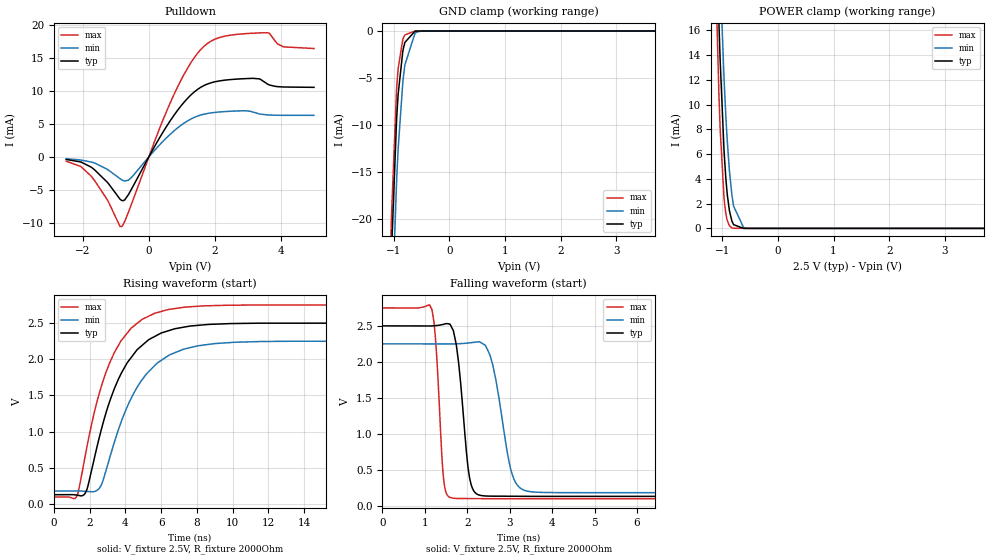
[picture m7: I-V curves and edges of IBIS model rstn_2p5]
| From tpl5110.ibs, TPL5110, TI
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|   Model
[Model]   rstn_2p5
Model_type   I/O_open_drain
Polarity   Non-Inverting
Enable   Active-Low
Vinl = 0.75
Vinh = 1.75
Vmeas = 1.25
Vref = 2.5
Cref = 1pF
Rref = 2000
|   typ   min   max
C_comp   0.474pF   0.343pF   0.582pF
[Voltage Range]   2.5   2.25   2.75
[Temperature Range]   25   105   -40
[Pullup Reference]   2.5   2.25   2.75
[Pulldown Reference]   0   0   0
[Power Clamp Reference]   2.5   2.25   2.75
[GND Clamp Reference]   0   0   0
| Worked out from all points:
|   slope of the pulldown table from 0 to 0.375 V, typ, clamps not added: 113 ohm
|   GND clamp passes 1 mA (typ) near -0.77 V on its own axis
|   POWER clamp passes 1 mA (typ) near -0.85 V on its own axis
|   falling waveform, V_fixture 2.5V, R_fixture 2000Ohm: 20-80 % time 217ps typ, 346ps min, 145ps max; typ from 2.5 V to 0.13 V
|   rising waveform, V_fixture 2.5V, R_fixture 2000Ohm: 20-80 % time 2.09ns typ, 2.26ns min, 1.95ns max; typ from 0.13 V to 2.5 V
[Pulldown]
|   Voltage   I(typ)   I(min)   I(max)
-2.5V     -377.8uA   -275.3uA   -643.7uA
-1.75V    -1.525mA   -756.3uA   -2.874mA
-827.5mV  -6.561mA   -3.438mA   -10.54mA
-512.5mV  -4.763mA   -3.037mA   -6.974mA
747.5mV   6.204mA    3.877mA    9.293mA
1.235V    9.192mA    5.639mA    13.95mA
1.67V     10.81mA    6.471mA    16.74mA
2.217V    11.57mA    6.84mA     18.18mA
3.147V    11.9mA     6.802mA    18.73mA
3.605V    10.99mA    6.358mA    18.79mA
4.077V    10.59mA    6.301mA    16.66mA
5V        10.54mA    6.298mA    16.41mA
[GND Clamp]
|   Voltage   I(typ)   I(min)   I(max)
-2.5V     -532.7mA   -498.3mA   -571.1mA
-1.045V   -24.97mA   -32.7mA    -21.13mA
-1.038V   -23.46mA   -31.2mA    -19.56mA
-947.5mV  -9.534mA   -16.15mA   -6.257mA
-940mV    -8.737mA   -15.16mA   -5.592mA
-917.5mV  -6.657mA   -12.44mA   -3.935mA
-835mV    -2.176mA   -5.473mA   -895.3uA
-820mV    -1.735mA   -4.645mA   -662.1uA
-797.5mV  -1.211mA   -3.602mA   -417uA
-617.5mV  -27.18uA   -264uA     -5.53uA
-512.5mV  -1.678uA   -25.84uA   -162.4nA
5V        0A         0A         0A
[POWER Clamp]
|   Voltage   I(typ)   I(min)   I(max)
-2.5V     351.8mA    332.8mA    370.5mA
-1.15V    31.09mA    37.5mA     25.49mA
-1.06V    16.49mA    23.38mA    10.69mA
-1.038V   13.47mA    20.27mA    7.946mA
-962.5mV  5.816mA    11.51mA    2.17mA
-910mV    2.716mA    7.028mA    631.3uA
-872.5mV  1.433mA    4.681mA    212.1uA
-827.5mV  591.6uA    2.703mA    43.28uA
-797.5mV  301.6uA    1.804mA    12.76uA
-617.5mV  1.108uA    70.67uA    0A
-565mV    156.4nA    19.84uA    0A
5V        0A         0A         0A
[Ramp]
R_load = 2000
|   typ   min   max
dV/dt_r   1.42208/2.09402e-09   1.24152/2.26178e-09   1.59152/1.95148e-09
dV/dt_f   1.42208/2.17249e-10   1.24152/3.46422e-10   1.59152/1.454e-10
[Falling Waveform]
V_fixture = 2.5V
V_fixture_min = 2.25V
V_fixture_max = 2.75V
R_fixture = 2000Ohm
C_fixture = 0F
|   Time   V(typ)   V(min)   V(max)
0s        2.5V       2.25V      2.75V
1.167ns   2.499V     2.249V     2.723V
1.281ns   2.505V     2.249V     2.05V
1.446ns   2.522V     2.249V     346.2mV
1.694ns   2.368V     2.249V     102.3mV
2.064ns   357mV      2.265V     99.11mV
2.428ns   135.2mV    2.228V     97.83mV
3.075ns   131.4mV    406mV      97.51mV
3.575ns   130mV      189.6mV    97.51mV
50ns      129.9mV    180.8mV    97.47mV
[Rising Waveform]
V_fixture = 2.5V
V_fixture_min = 2.25V
V_fixture_max = 2.75V
R_fixture = 2000Ohm
C_fixture = 0F
|   Time   V(typ)   V(min)   V(max)
0s        129.9mV    180.8mV    97.47mV
1.309ns   124mV      181.5mV    120.6mV
1.843ns   195.3mV    175mV      779.9mV
2.535ns   912.1mV    215.4mV    1.523V
3.192ns   1.466V     695.6mV    1.986V
4.104ns   1.951V     1.343V     2.361V
5.195ns   2.246V     1.802V     2.581V
6.404ns   2.393V     2.049V     2.687V
11.55ns   2.498V     2.244V     2.749V
50ns      2.5V       2.25V      2.75V
